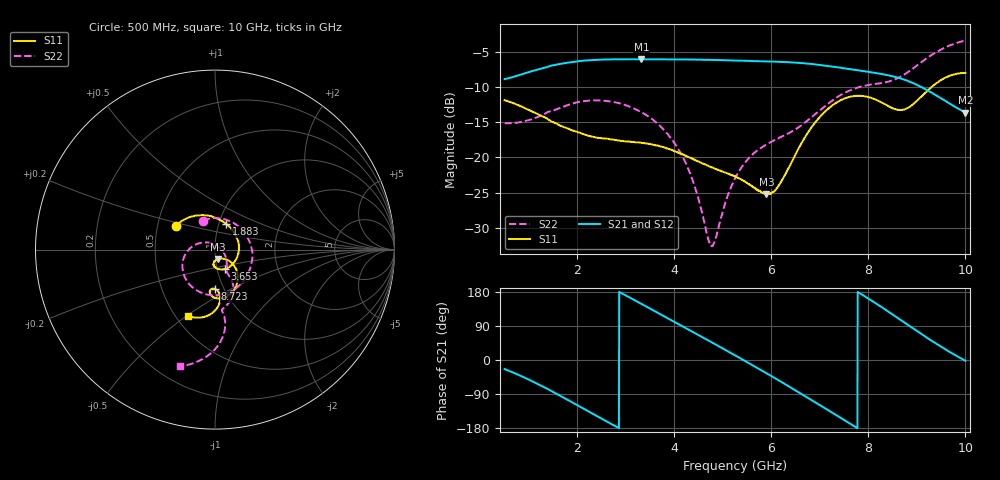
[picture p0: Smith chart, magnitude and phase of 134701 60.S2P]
!  2-Port S-parameters saved by WinCal
! VAR MeasName=S-Parameters (CALIBRATED_DATA) read from VNA (N5242A)
! VAR MeasDate=2013-7-3 16:41:04
! VAR NAME=134701 60
! VAR FILENAME=134701 60.S2P
! VAR DATE=2013-7-3 16:41:04
! VAR PHYS_PORTS=1,2
# Hz S MA R 50
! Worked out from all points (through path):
!   1601 points, 500 MHz to 10 GHz, reference 50 ohm
!   highest |S21| = -6.05 dB at 3.32 GHz (marker M1); lowest = -13.6 dB at 10 GHz (marker M2)
!   group delay of S21, straight-line fit = 205 ps
!   lowest |S11| = -25.2 dB at 5.897 GHz (marker M3), VSWR 1.12, Z = 51.2 - j5.42 ohm
!   |S11| at or under -10 dB: start of sweep to 9.302 GHz
!   |S22| runs from -32.6 to -3.4 dB; largest |S21 - S12| = 0.002
!   S11 on the Smith chart (normalised r, x): 500 MHz: 0.62, +0.18; 1.883 GHz: 1.08, +0.32; 3.653 GHz: 1.09, -0.24; 8.723 GHz: 0.91, -0.42; 10 GHz: 0.57, -0.50
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5e8  0.2552 148.9  0.3601 -24.0  0.3596 -24.0  0.175 112.4
8.5625e8  0.2293 127.8  0.3901 -43.3  0.3898 -43.3  0.179 62.7
1.26e9  0.1972 104.5  0.4283 -68.4  0.4286 -68.3  0.1987 10.1
1.883438e9  0.1563 66.7  0.4756 -111.2  0.4762 -111.2  0.24 -54.2
2.085312e9  0.1482 52.5  0.4852 -125.4  0.4854 -125.5  0.2498 -71.1
2.714688e9  0.134 3.5  0.4969 -169.9  0.4975 -170.0  0.2485 -114.8
3.320312e9  0.1273 -41.9  0.4985 148.0  0.498 148.0  0.2093 -149.7
3.652812e9  0.1216 -62.4  0.4978 125.0  0.4977 125.0  0.1738 -168.1
3.670625e9  0.121 -63.5  0.4984 123.8  0.4972 123.7  0.1715 -169.1
4.2525e9  0.1018 -87.6  0.4964 83.1  0.4965 83.2  0.08858 154.9
4.757188e9  0.08536 -95.7  0.4933 47.5  0.4935 47.5  0.02383 62.4
5.25e9  0.07341 -95.8  0.4878 12.2  0.4883 12.2  0.07101 -33.6
5.897188e9  0.05483 -74.2  0.4809 -34.8  0.4813 -34.8  0.1233 -58.8
6.39e9  0.08842 -39.8  0.474 -71.8  0.4747 -71.9  0.1507 -62.1
6.835312e9  0.1649 -43.7  0.461 -106.3  0.4615 -106.3  0.1934 -61.6
7.262812e9  0.2353 -60.0  0.4415 -139.7  0.4425 -139.7  0.2546 -66.4
7.636875e9  0.2705 -76.4  0.4229 -169.2  0.424 -169.2  0.3012 -74.3
8.016875e9  0.2673 -90.8  0.4047 160.6  0.405 160.5  0.3274 -81.3
8.420625e9  0.2306 -97.1  0.3825 126.8  0.3823 126.7  0.3462 -83.4
8.723438e9  0.2182 -90.4  0.3581 100.5  0.3589 100.4  0.3852 -82.0
9.335e9  0.3233 -87.7  0.2839 47.9  0.2847 47.8  0.5431 -88.9
1e10  0.3986 -112.5  0.208 -2.1  0.2083 -2.4  0.6777 -106.6
